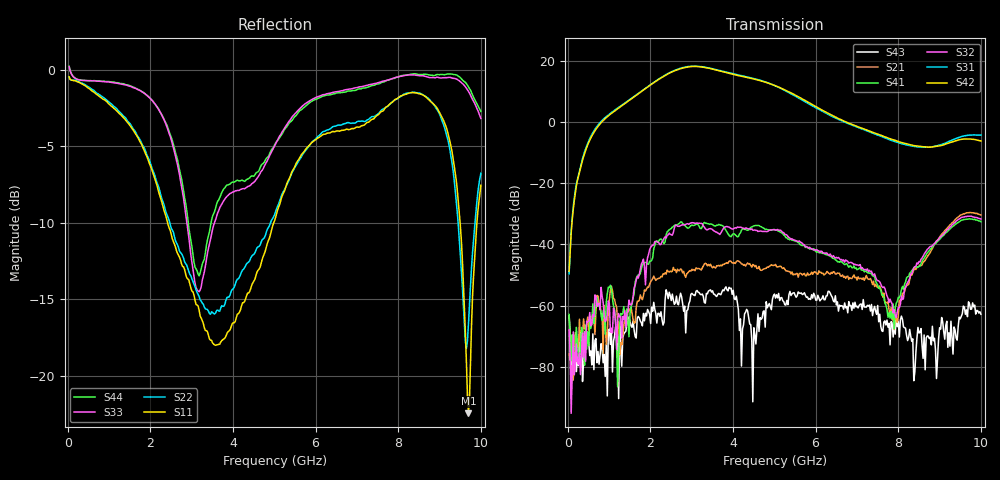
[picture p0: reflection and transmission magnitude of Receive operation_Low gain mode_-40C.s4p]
! Device:  ADRF5545A
! Description: Dual-Channel, Receiver Front End
! Frequency:  2.4 -  4.2 GHz
! Ports:
!	ANT-CHA	= Port 1
!	ANT-CHB	= Port 2
!  RXOUT-CHA = Port 3
!	RXOUT-CHB = Port 4
! VDD1-CHA, VDD1-CHB, VDD2-CHA, VDD2-CHB, and SWVDD-CHAB = 5 V
! SWCTRL-CHAB = 0 V,  PD-CHAB = 0 V,BP-CHA=BP-CHB=5V
! Temp=-40C
! Data:  Data was collected using a calibrated 4 port network analyzer and de-embedded using AtaiTec's In Situ De-Embedding.
! Note:  Analog Devices supplies this data as a sample of measured data
!  for this product.  Your particular data for this product may vary.
!  Data was taken at -40 degrees C.
!  Analog Devices reserves the right to change this data at anytime.
!Correction: S11(Full 4 Port(1,2,3,4))
!S12(Full 4 Port(1,2,3,4))
!S13(Full 4 Port(1,2,3,4))
!S14(Full 4 Port(1,2,3,4))
!S21(Full 4 Port(1,2,3,4))
!S22(Full 4 Port(1,2,3,4))
!S23(Full 4 Port(1,2,3,4))
!S24(Full 4 Port(1,2,3,4))
!S31(Full 4 Port(1,2,3,4))
!S32(Full 4 Port(1,2,3,4))
!S33(Full 4 Port(1,2,3,4))
!S34(Full 4 Port(1,2,3,4))
!S41(Full 4 Port(1,2,3,4))
!S42(Full 4 Port(1,2,3,4))
!S43(Full 4 Port(1,2,3,4))
!S44(Full 4 Port(1,2,3,4))
!S4P File: Measurements: <S11,S12,S13,S14>,
!<S21,S22,S23,S24>,
!<S31,S32,S33,S34>,
!<S41,S42,S43,S44>:
# Hz S  dB  R 50
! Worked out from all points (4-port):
!   400 points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, 34.98 MHz to 10 GHz, reference 50 ohm
!   strongest paths, dB at 34.98 MHz, 2.532 GHz, 5.03 GHz, 7.527 GHz, 10 GHz:
!     S42: -48.8, 16.3, 11.7, -4.1, -6.3
!     S31: -49.6, 16.5, 11.7, -4.5, -4.4
!     S32: -67.9, -37.0, -35.3, -51.9, -31.7
!     S41: -62.9, -34.4, -35.4, -54.3, -32.6
!     S21: -75.8, -48.7, -46.6, -54.1, -30.4
!     S43: -63.3, -56.2, -57.5, -65.3, -62.8
!   lowest |S11| = -22.5 dB at 9.7 GHz (marker M1), VSWR 1.16, Z = 44.3 + j4.24 ohm
!   |S11| at or under -10 dB: 2.417 GHz to 4.989 GHz (2.571 GHz wide, 69.4 % of centre); 9.497 GHz to 9.904 GHz (406.7 MHz wide, 4.19 % of centre)
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3.4975e7  -0.46 -11.3  -71.15 136.1  -63.91 -147.1  -67.32 79.2
          -75.75 17.1  -0.49 -11.2  -62.95 94.6  -59.50 -76.4
          -49.59 -1.3  -67.91 -51.5  0.20 -7.1  -65.27 -87.8
          -62.87 176.1  -48.75 2.3  -63.30 117.0  0.23 -7.1
2.182825e9  -7.80 -155.7  -50.57 90.7  -44.41 120.2  -73.12 158.4
            -51.22 92.4  -7.55 -161.4  -67.47 149.2  -44.50 118.4
            13.77 137.4  -39.32 49.2  -2.52 -108.0  -56.58 138.1
            -39.19 65.8  13.64 136.8  -62.54 126.2  -2.49 -108.6
3.25675e9  -16.40 43.4  -47.37 37.1  -34.20 7.3  -74.29 30.7
           -47.74 40.0  -15.26 36.0  -71.67 42.1  -34.63 6.0
           17.97 6.4  -33.28 -100.9  -13.78 -101.5  -55.75 79.6
           -34.32 -75.3  17.87 5.1  -56.20 76.1  -12.70 -104.3
3.95605e9  -16.81 -9.3  -46.47 13.2  -33.44 -56.2  -66.84 32.7
           -45.58 0.5  -14.50 -5.3  -75.73 -32.5  -34.02 -57.1
           15.84 -66.2  -34.80 -153.5  -8.07 -110.3  -54.56 25.7
           -37.49 -153.5  15.63 -67.5  -54.32 5.5  -7.40 -104.9
4.85515e9  -11.18 33.5  -45.26 -21.1  -33.62 -131.4  -65.66 3.7
           -47.48 -24.3  -10.33 29.7  -76.28 -95.1  -33.98 -130.7
           12.68 -150.6  -35.64 128.2  -5.81 159.8  -78.39 53.6
           -35.25 127.5  12.61 -151.3  -59.93 97.9  -5.68 169.6
9.7003e9  -22.46 140.8  -30.15 -143.2  -42.17 34.8  -57.20 51.4
          -29.66 -144.3  -16.59 150.0  -61.46 -13.9  -43.03 24.6
          -4.37 -42.1  -30.84 -118.0  -1.42 79.9  -57.86 13.9
          -31.72 -106.0  -5.59 -52.4  -58.75 -9.2  -1.13 78.0
1e10  -7.56 -154.3  -30.99 165.5  -42.00 12.2  -56.23 44.4
      -30.41 164.6  -6.77 174.8  -65.22 15.6  -43.54 -1.6
      -4.35 -75.0  -31.73 -171.6  -3.18 75.5  -59.94 -5.4
      -32.61 -159.8  -6.26 -83.3  -62.80 -18.5  -2.73 75.3
